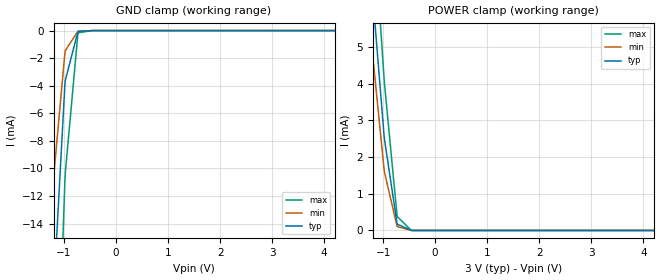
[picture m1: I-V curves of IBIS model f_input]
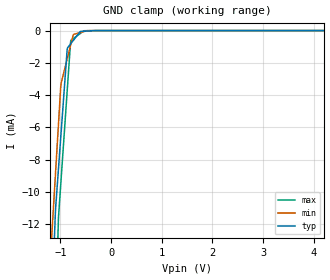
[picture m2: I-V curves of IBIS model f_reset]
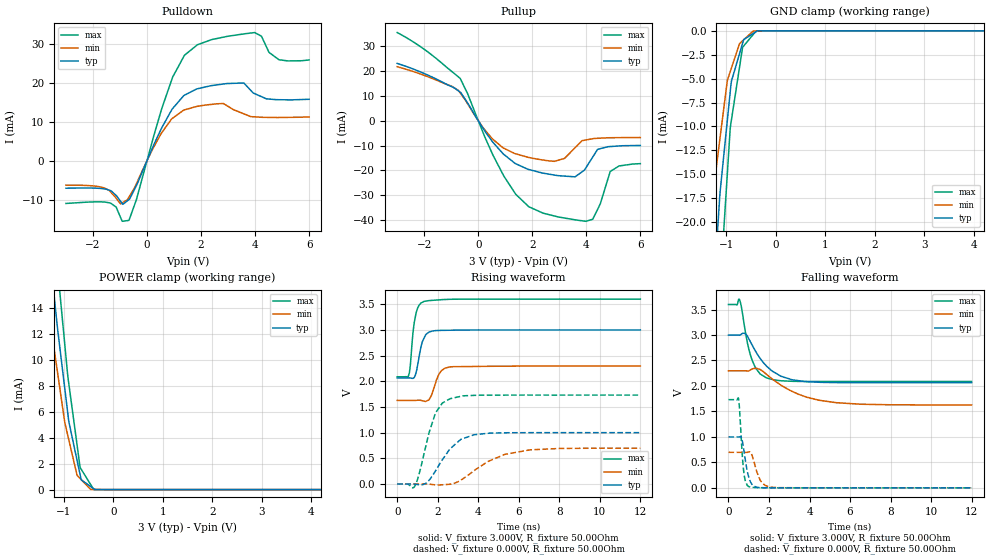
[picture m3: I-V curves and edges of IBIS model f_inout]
[IBIS Ver]   3.2
[File Name]   rc_p33_30v_64m_b.ibs
[File Rev]   1.01
[Date]   3/10/2010
[Source]   From silicon level SPICE model at Numonyx B.V.
[Notes]   The following information corresponds to the
   Redcliff 65nm P33 64Mb chip with EZBGA package.
[Disclaimer]   This information is for modeling purposes only and is not
   guaranteed.Numonyx B.V. is not responsible for any problem
   this model may cause to customers.
[Copyright]   Copyright 2010, Numonyx B.V., All Rights Reserved.
[Component]   P33_30V_64M_EZBGA
[Manufacturer]  Numonyx B.V.
[Package]
|   typ   min   max
R_pkg   0.33Ohm   0.16Ohm   0.50Ohm
L_pkg   6.69nH   3.42nH   9.96nH
C_pkg   1.25pF   0.27pF   2.23pF
[PIN]   signal_name   model_name   R_pin   L_pin   C_pin
A1   A1   f_input   0.28   5.77nH   0.65pF
A2   A6   f_input   0.36   7.41nH   0.92pF
A3   A8   f_input   0.20   4.23nH   0.40pF
A4   NC   NC
A5   A13   f_input   0.16   3.42nH   0.27pF
A6   VCC   POWER
A7   A18   f_input   0.26   5.74nH   0.67pF
A8   A22   f_input   0.33   7.38nH   0.83pF
B1   A2   f_input   0.27   5.51nH   0.60pF
B2   VSS   GND
B3   A9   f_input   0.35   7.25nH   0.89pF
B4   CE#   f_input   0.43   8.13nH   1.28pF
B5   A14   f_input   0.23   4.66nH   0.46pF
B6   NC   NC
B7   A19   f_input   0.26   5.62nH   0.64pF
B8   NC   NC
C1   A3   f_input   0.29   5.77nH   0.64pF
C2   A7   f_input   0.29   5.73nH   0.64pF
C3   A10   f_input   0.35   7.03nH   0.85pF
C4   A12   f_input   0.34   6.86nH   0.82pF
C5   A15   f_input   0.27   5.44nH   0.59pF
C6   WP#   f_input   0.27   5.44nH   0.59pF
C7   A20   f_input   0.41   8.27nH   1.06pF
C8   A21   f_input   0.33   6.76nH   0.81pF
D1   A4   f_input   0.30   6.07nH   0.69pF
D2   A5   f_input   0.28   5.47nH   0.59pF
D3   A11   f_input   0.37   7.50nH   0.93pF
D4   RST#   f_reset   0.32   6.25nH   0.83pF
D5   VCCQ   POWER
D6   VCCQ   POWER
D7   A16   f_input   0.25   4.83nH   0.48pF
D8   A17   f_input   0.29   5.71nH   0.62pF
E1   DQ8   f_inout   0.28   6.28nH   0.82pF
E2   DQ1   f_inout   0.26   5.20nH   0.63pF
E3   DQ9   f_inout   0.25   4.92nH   0.56pF
E4   DQ3   f_inout   0.25   4.98nH   0.58pF
E5   DQ4   f_inout   0.30   5.87nH   0.65pF
E6   CLK   f_input   0.29   5.72nH   0.73pF
E7   DQ15   f_inout   0.27   5.36nH   0.56pF
E8   NC   NC
F1   NC   NC
F2   DQ0   f_inout   0.21   4.33nH   0.46pF
F3   DQ10   f_inout   0.23   4.69nH   0.55pF
F4   DQ11   f_inout   0.23   4.60nH   0.52pF
F5   DQ12   f_inout   0.20   4.02nH   0.43pF
F6   ADV#   f_input   0.25   4.85nH   0.49pF
F7   WAIT   f_inout   0.24   4.71nH   0.53pF
F8   OE#   f_input   0.42   9.70nH   2.23pF
G1   NC   NC
G2   NC   NC
G3   DQ2   f_inout   0.22   4.43nH   0.42pF
G4   VCCQ   POWER
G5   DQ5   f_inout   0.17   3.51nH   0.35pF
G6   DQ6   f_inout   0.18   3.76nH   0.40pF
G7   DQ14   f_inout   0.22   4.44nH   0.42pF
G8   WE#   f_input   0.50   9.96nH   1.33pF
H1   NC   NC
H2   VSS   GND
H3   VCC   POWER
H4   VSS   GND
H5   DQ13   f_inout   0.21   4.31nH   0.41pF
H6   VSSQ   GND
H7   DQ7   f_inout   0.23   4.67nH   0.46pF
H8   NC   NC
| Models and submodels in the file (3): f_input (Input), f_reset (Input), f_inout (I/O)
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[Model]   f_input
Model_type   Input
Vinl = 0.400V
Vinh = 2.600V
|   typ   min   max
C_comp   6.000pF   2.000pF   7.000pF
[Voltage Range]   3.000V   2.300V   3.600V
[Temperature Range]   25.0   85.0   -40.0
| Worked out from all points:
|   GND clamp passes 1 mA (typ) near -0.79 V on its own axis
|   POWER clamp passes 1 mA (typ) near -0.82 V on its own axis
[GND Clamp]
|   Voltage   I(typ)   I(min)   I(max)
-3V       -214.2mA   -171.1mA   -282mA
-1.398V   -38.01mA   -24.9mA    -60.4mA
-1.209V   -20.02mA   -11.33mA   -36.27mA
-1.2V     -19.19mA   -10.72mA   -35.15mA
-984mV    -4.085mA   -1.721mA   -11.16mA
-975mV    -3.631mA   -1.46mA    -10.38mA
-732mV    -88.55uA   -49.57uA   -226.8uA
-723mV    -64.96uA   -39.8uA    -159.9uA
-453mV    -377.4nA   -554.6nA   -216.8nA
6V        0A         0A         0A
[POWER Clamp]
|   Voltage   I(typ)   I(min)   I(max)
-3V       44.58mA    39.22mA    51.64mA
-1.299V   8.339mA    6.46mA     11.02mA
-1.209V   6.572mA    4.919mA    8.979mA
-1.2V     6.398mA    4.769mA    8.776mA
-984mV    2.624mA    1.697mA    4.188mA
-975mV    2.493mA    1.595mA    4.017mA
-732mV    187.3uA    115.4uA    401uA
-723mV    168.4uA    103.4uA    368.4uA
-453mV    1.105uA    1.525uA    700.3nA
6V        0A         0A         0A
[Model]   f_reset
Model_type   Input
Vinl = 0.400V
Vinh = 2.600V
|   typ   min   max
C_comp   6.000pF   2.000pF   7.000pF
[Voltage Range]   3.000V   2.300V   3.600V
[Temperature Range]   25.0   85.0   -40.0
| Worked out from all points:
|   GND clamp passes 1 mA (typ) near -0.84 V on its own axis
[GND Clamp]
|   Voltage   I(typ)   I(min)   I(max)
-3V       -205.4mA   -173mA     -256.3mA
-1.209V   -20.5mA    -14.72mA   -29.6mA
-1.101V   -11.42mA   -9.082mA   -18.23mA
-1.047V   -8.959mA   -6.264mA   -12.54mA
-1.038V   -8.571mA   -5.795mA   -11.6mA
-993mV    -6.627mA   -3.447mA   -9.54mA
-867mV    -1.187mA   -1.777mA   -3.783mA
-795mV    -811.6uA   -873.4uA   -609.4uA
-741mV    -594.7uA   -238.1uA   -486.6uA
-606mV    -54.38uA   -121.6uA   -179.4uA
-318mV    -41.02nA   -2.805uA   -2.579uA
6V        0A         0A         0A
[POWER Clamp]
|   Voltage   I(typ)   I(min)   I(max)
-3V       0A         0A         0A
0V        0A         0A         0A
2.301V    0A         0A         0A
3.003V    0A         0A         0A
3.597V    0A         0A         0A
6V        0A         0A         0A
[Model]   f_inout
Model_type   I/O
Vinl = 0.400V
Vinh = 2.600V
Vmeas = 1.500V
Cref = 30.0pF
|   typ   min   max
C_comp   4.000pF   2.000pF   5.000pF
[Voltage Range]   3.000V   2.300V   3.600V
[Temperature Range]   25.0   85.0   -40.0
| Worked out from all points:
|   slope of the pulldown table from 0 to 0.45 V, typ, clamps not added: 64.1 ohm
|   slope of the pullup table from 0 to 0.45 V, typ, clamps not added: 61.5 ohm
|   GND clamp passes 1 mA (typ) near -0.65 V on its own axis
|   POWER clamp passes 1 mA (typ) near -0.66 V on its own axis
|   falling waveform, V_fixture 3.000V, R_fixture 50.00Ohm: 20-80 % time 1.18ns typ, 1.97ns min, 555ps max; typ from 3 V to 2.06 V
|   rising waveform, V_fixture 3.000V, R_fixture 50.00Ohm: 20-80 % time 312ps typ, 381ps min, 252ps max; typ from 2.06 V to 3 V
|   rising waveform, V_fixture 0.000V, R_fixture 50.00Ohm: 20-80 % time 1.14ns typ, 1.81ns min, 713ps max; typ from 0.001 V to 1 V
|   falling waveform, V_fixture 0.000V, R_fixture 50.00Ohm: 20-80 % time 274ps typ, 357ps min, 175ps max; typ from 1 V to 0.001 V
[Pulldown]
|   Voltage   I(typ)   I(min)   I(max)
-3V       -7.107mA   -6.316mA   -11.01mA
-1.353V   -7.712mA   -8.02mA    -10.92mA
-975mV    -10.52mA   -11.1mA    -14.67mA
-669mV    -10.02mA   -9.382mA   -15.34mA
942mV     13.28mA    10.83mA    21.27mA
1.383V    16.74mA    12.98mA    26.95mA
1.869V    18.41mA    13.91mA    29.71mA
2.823V    19.62mA    14.63mA    31.63mA
3.579V    19.89mA    11.99mA    32.47mA
3.984V    17.15mA    11.2mA     32.82mA
4.884V    15.6mA     11.04mA    25.85mA
6V        15.71mA    11.17mA    25.8mA
[GND Clamp]
|   Voltage   I(typ)   I(min)   I(max)
-3V       -194mA     -149mA     -233.1mA
-1.326V   -32.85mA   -21.96mA   -46.85mA
-1.2V     -22.84mA   -14.26mA   -34.15mA
-1.146V   -18.54mA   -12.06mA   -28.71mA
-1.119V   -16.59mA   -10.95mA   -26.46mA
-984mV    -9.685mA   -5.433mA   -15.45mA
-921mV    -6.464mA   -4.302mA   -10.32mA
-894mV    -5.245mA   -3.88mA    -9.284mA
-732mV    -2.399mA   -1.35mA    -3.827mA
-669mV    -1.293mA   -1.037mA   -1.718mA
-453mV    -276.2uA   -31.54uA   -368.6uA
6V        0A         0A         0A
[Pullup]
|   Voltage   I(typ)   I(min)   I(max)
-3V       23.17mA    21.83mA    35.6mA
-669mV    11.57mA    11.27mA    17.11mA
186mV     -3.134mA   -2.881mA   -4.963mA
951mV     -13.57mA   -11.07mA   -22.35mA
1.869V    -19.62mA   -14.76mA   -34.62mA
2.823V    -21.86mA   -16.32mA   -38.37mA
3.579V    -22.57mA   -10.89mA   -39.89mA
3.93V     -19.86mA   -7.806mA   -40.42mA
4.236V    -14.61mA   -7.204mA   -39.69mA
4.515V    -11.22mA   -6.979mA   -33.53mA
4.884V    -10.36mA   -6.807mA   -20.42mA
6V        -9.919mA   -6.716mA   -17.26mA
[POWER Clamp]
|   Voltage   I(typ)   I(min)   I(max)
-3V       90.42mA    73.44mA    106.8mA
-1.326V   19.74mA    14.81mA    25.76mA
-1.2V     15.13mA    10.98mA    20.25mA
-1.119V   12.19mA    8.85mA     16.79mA
-984mV    7.942mA    5.302mA    11.37mA
-903mV    5.391mA    3.918mA    8.301mA
-732mV    2.27mA     1.12mA     3.471mA
-669mV    1.141mA    853.4uA    1.702mA
-642mV    742.5uA    747.1uA    1.535mA
-453mV    228.5uA    14.79uA    368.9uA
-390mV    57.19uA    11.69uA    6.143uA
6V        0A         0A         0A
[Ramp]
R_load = 50.00Ohm
|   typ   min   max
dV/dt_r   599.255mV/1.138ns   417.739mV/1.812ns   1.038V/713.059ps
dV/dt_f   560.609mV/1.176ns   401.891mV/1.974ns   906.641mV/554.749ps
[Falling Waveform]
V_fixture = 3.000V
V_fixture_min = 2.300V
V_fixture_max = 3.600V
R_fixture = 50.00Ohm
|   Time   V(typ)   V(min)   V(max)
0s        2.998V     2.297V     3.598V
420ps     2.998V     2.297V     3.591V
540ps     2.996V     2.297V     3.7V
840ps     3.021V     2.297V     3.044V
1.17ns    2.8V       2.334V     2.502V
1.56ns    2.543V     2.323V     2.236V
1.89ns    2.385V     2.224V     2.157V
3.14ns    2.121V     1.894V     2.092V
4.48ns    2.072V     1.719V     2.088V
12ns      2.064V     1.627V     2.087V
[Rising Waveform]
V_fixture = 3.000V
V_fixture_min = 2.300V
V_fixture_max = 3.600V
R_fixture = 50.00Ohm
|   Time   V(typ)   V(min)   V(max)
0s        2.064V     1.627V     2.087V
540ps     2.065V     1.627V     2.089V
640ps     2.065V     1.627V     2.29V
780ps     2.057V     1.627V     2.955V
930ps     2.17V      1.628V     3.327V
1.33ns    2.845V     1.612V     3.556V
1.57ns    2.955V     1.64V      3.57V
2.18ns    2.991V     2.206V     3.588V
2.6ns     2.993V     2.279V     3.595V
12ns      2.998V     2.297V     3.598V
[Rising Waveform]
V_fixture = 0.000V
V_fixture_min = 0.000V
V_fixture_max = 0.000V
R_fixture = 50.00Ohm
|   Time   V(typ)   V(min)   V(max)
0s        751.6uV    1.671mV    724.9uV
840ps     -1.594mV   1.564mV    -59.79mV
1.07ns    -12.51mV   1.971mV    181.7mV
1.4ns     9.498mV    2.359mV    718.6mV
1.88ns    249.9mV    -15.83mV   1.375V
2.61ns    685.5mV    -3.42mV    1.661V
3.79ns    959.5mV    258.4mV    1.725V
5.31ns    996.9mV    576.9mV    1.731V
8.03ns    999.5mV    692.3mV    1.731V
12ns      999.5mV    697.9mV    1.731V
[Falling Waveform]
V_fixture = 0.000V
V_fixture_min = 0.000V
V_fixture_max = 0.000V
R_fixture = 50.00Ohm
|   Time   V(typ)   V(min)   V(max)
0s        999.5mV    697.9mV    1.731V
490ps     999.3mV    697.9mV    1.761V
540ps     999.2mV    697.9mV    1.58V
640ps     983.2mV    697.9mV    908.4mV
740ps     787.3mV    697.9mV    364.7mV
840ps     524.4mV    697.6mV    124.1mV
1.01ns    199.6mV    706.9mV    23.72mV
1.57ns    4.802mV    146.8mV    4.154mV
2.06ns    1.815mV    17.75mV    1.706mV
12ns      751.6uV    1.671mV    724.9uV
